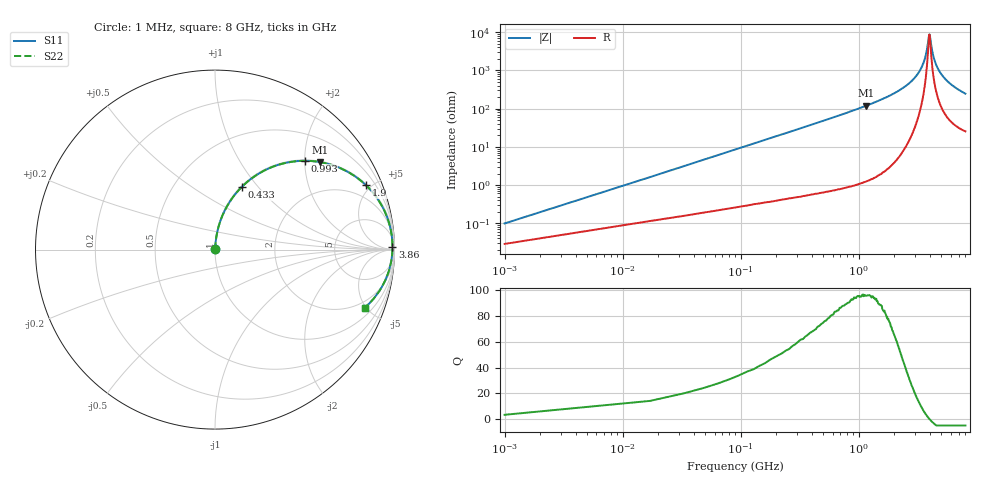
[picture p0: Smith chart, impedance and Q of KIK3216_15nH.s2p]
!version-2
!date-01.2022
!Series
# MHz S RI R 50
!Freq ReS11 ImS11 ReS21 ImS21 ReS12 ImS12 ReS22 ImS22
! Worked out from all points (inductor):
!   501 points, 1 MHz to 8 GHz, reference 50 ohm
!   read as one part in series: L = 15 nH near 33 MHz
!   highest Q = 96.1 at 1.15 GHz (marker M1), where L = 16.4 nH
!   self-resonance near 3.97 GHz
!   S11 on the Smith chart (normalised r, x): 1 MHz: 1.00, +0.00; 433 MHz: 1.01, +0.83; 993 MHz: 1.02, +2.00; 1.9 GHz: 1.07, +4.67; 3.86 GHz: open; 8 GHz: 1.51, -4.90
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1  0.000275 0.000942  0.9997 -0.000942  0.9997 -0.000942  0.000275 0.000942
49  0.00404 0.0459  0.996 -0.0459  0.996 -0.0459  0.00404 0.0459
97  0.0109 0.0902  0.9891 -0.0902  0.9891 -0.0902  0.0109 0.0902
225  0.0469 0.2019  0.9531 -0.2019  0.9531 -0.2019  0.0469 0.2019
433  0.1493 0.3493  0.8507 -0.3493  0.8507 -0.3493  0.1493 0.3493
993  0.4992 0.4948  0.5008 -0.4948  0.5008 -0.4948  0.4992 0.4948
1150  0.584 0.4877  0.416 -0.4877  0.416 -0.4877  0.584 0.4877
1340  0.6706 0.4647  0.3294 -0.4647  0.3294 -0.4647  0.6706 0.4647
1900  0.8413 0.3584  0.1587 -0.3584  0.1587 -0.3584  0.8413 0.3584
2670  0.9491 0.2044  0.0509 -0.2044  0.0509 -0.2044  0.9491 0.2044
3140  0.9764 0.1229  0.0236 -0.1229  0.0236 -0.1229  0.9764 0.1229
3460  0.9855 0.0724  0.0145 -0.0724  0.0145 -0.0724  0.9855 0.0724
3700  0.9884 0.0372  0.0116 -0.0372  0.0116 -0.0372  0.9884 0.0372
3860  0.9889 0.0151  0.0111 -0.0151  0.0111 -0.0151  0.9889 0.0151
3950  0.9887 0.00224  0.0113 -0.00224  0.0113 -0.00224  0.9887 0.00224
4020  0.9884 -0.00614  0.0116 0.00614  0.0116 0.00614  0.9884 -0.00614
4190  0.9868 -0.0284  0.0132 0.0284  0.0132 0.0284  0.9868 -0.0284
4430  0.983 -0.0572  0.0169 0.0572  0.0169 0.0572  0.983 -0.0572
4780  0.975 -0.0961  0.025 0.0961  0.025 0.0961  0.975 -0.0961
5350  0.9572 -0.1511  0.0428 0.1511  0.0428 0.1511  0.9572 -0.1511
6670  0.9004 -0.2528  0.0996 0.2528  0.0996 0.2528  0.9004 -0.2528
8000  0.8346 -0.3233  0.1654 0.3233  0.1654 0.3233  0.8346 -0.3233
